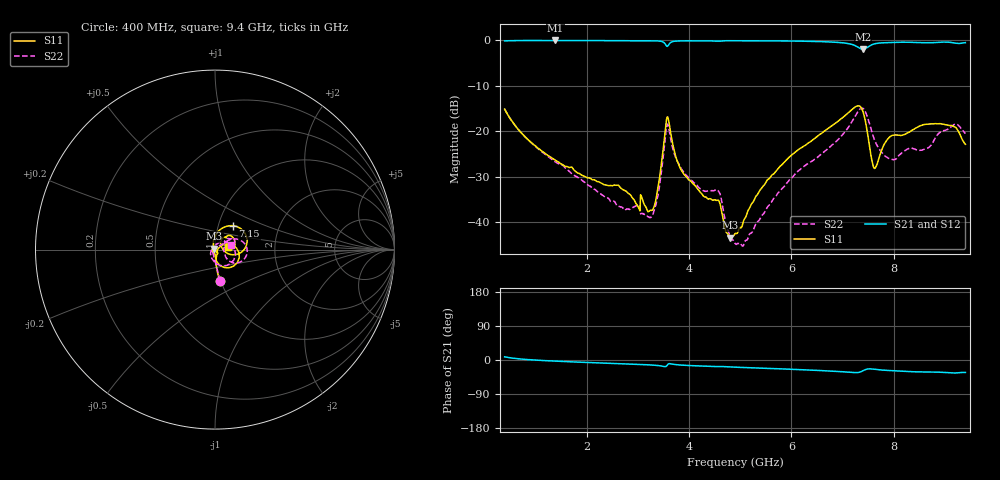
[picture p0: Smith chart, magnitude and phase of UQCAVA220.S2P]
!  Part Number  UQCAVA220 Mounting Orientation: Vertical
!  Description: RF capacitors
!  Application: Coupling, Bypass, Tuning, DC Block
!  Filters, Matching
# GHZ S DB R 50
! Freq  |S11|  S11 Ph  |S21|  S21 Ph  |S12|  S12 Ph  |S22|  S22 Ph
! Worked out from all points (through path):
!   801 points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, 400 MHz to 9.4 GHz, reference 50 ohm
!   highest |S21| = -0.07 dB at 1.39 GHz (marker M1); lowest = -2.0 dB at 7.398 GHz (marker M2)
!   group delay of S21, straight-line fit = 11.5 ps
!   lowest |S11| = -43.4 dB at 4.81 GHz (marker M3), VSWR 1.01, Z = 49.7 + j0.604 ohm
!   |S11| at or under -10 dB: start of sweep to end of sweep
!   |S22| runs from -45.2 to -14.9 dB; largest |S21 - S12| = 0.0074
!   S11 on the Smith chart (normalised r, x): 400 MHz: 0.99, -0.35; 7.15 GHz: 1.18, +0.32; 9.4 GHz: 1.15, +0.03
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0.4  -15.13 -81.2  -0.17 8.4  -0.14 8.4  -15.10 -80.1
1.39  -26.33 -83.0  -0.07 -3.0  -0.04 -3.1  -26.70 -93.8
1.908  -29.63 -74.0  -0.09 -6.0  -0.05 -6.1  -30.72 -108.3
2.616  -31.82 -52.3  -0.13 -9.7  -0.10 -9.8  -36.41 -158.4
3.235  -37.38 -25.2  -0.14 -12.9  -0.11 -13.1  -38.88 130.9
3.404  -31.83 26.1  -0.18 -14.8  -0.15 -14.9  -33.58 89.3
3.55  -18.37 3.5  -1.07 -17.1  -1.04 -17.3  -20.06 13.3
3.595  -17.15 -41.4  -1.19 -10.8  -1.16 -10.9  -18.68 -42.2
3.876  -28.97 -86.2  -0.16 -13.7  -0.14 -13.8  -28.63 -130.6
4.574  -35.12 -164.2  -0.24 -17.3  -0.22 -17.6  -33.07 163.9
4.81  -43.36 116.5  -0.12 -18.4  -0.10 -18.6  -43.36 132.9
4.9  -42.45 109.9  -0.12 -18.9  -0.11 -19.1  -44.58 126.2
5.091  -39.11 114.2  -0.13 -20.0  -0.11 -20.2  -44.22 98.8
5.541  -30.57 106.6  -0.18 -22.2  -0.17 -22.4  -36.49 53.3
6.408  -21.97 87.7  -0.28 -26.9  -0.28 -27.1  -26.53 36.0
7.15  -15.56 52.9  -0.84 -32.5  -0.85 -32.8  -18.51 29.8
7.398  -15.62 1.6  -2.03 -28.5  -2.04 -28.8  -14.96 -9.3
7.623  -28.15 20.4  -0.82 -24.4  -0.84 -24.7  -21.81 -37.2
7.904  -21.44 53.7  -0.54 -27.6  -0.56 -28.0  -25.94 -9.2
8.658  -18.43 36.8  -0.57 -31.7  -0.59 -32.0  -23.71 34.0
8.916  -18.35 25.2  -0.46 -32.3  -0.49 -32.6  -20.16 38.4
9.4  -22.85 9.8  -0.55 -32.8  -0.58 -33.1  -20.49 16.8
